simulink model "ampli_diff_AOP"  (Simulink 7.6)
settings: Solver=ode45  StartTime=0.0  StopTime=10.0  RelTol=1e-3
undefined symbols (not defined in the file or in its folder): Rb
libraries: fl_lib x16, nesl_utility x3

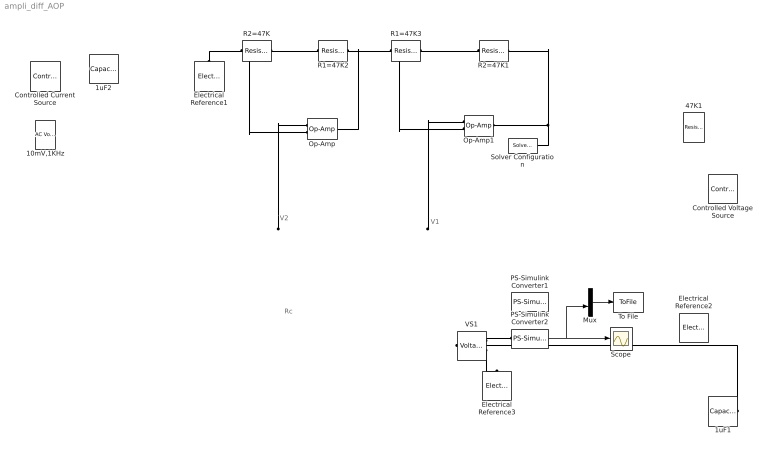
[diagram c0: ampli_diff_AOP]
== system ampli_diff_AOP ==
  note: Rc
  note: V2
  note: V1
  10mV,1KHz : fl_lib/Electrical/Electrical Sources/AC Voltage Source  DialogController=NetworkEngine.DynNeDlgSource  SystemSampleTime=-1  amp=0.01 V  shift=0 rad  omega=1000 Hz  i_Log=off  v_Log=off  LocalVarNames=|current|voltage|power  LocalVarDescs=|Current (A)|Voltage (V)|Power (W)  LocalVarLogging=[0 0 0]
  1uF1 : fl_lib/Electrical/Electrical Elements/Capacitor  DialogController=NetworkEngine.DynNeDlgSource  SystemSampleTime=-1  c=1e-06 F  v0=0 V  r=1e-06 Ohm  g=0 1/Ohm  i_Log=off  v_Log=off  vc_Log=off  LocalVarNames=|current|voltage|power  LocalVarDescs=|Capacitor current (A)|Voltage across capacitor (V)|Power (W)  LocalVarLogging=[0 0 0]
  1uF2 : fl_lib/Electrical/Electrical Elements/Capacitor  DialogController=NetworkEngine.DynNeDlgSource  SystemSampleTime=-1  c=1e-06 F  v0=0 V  r=1e-06 Ohm  g=0 1/Ohm  i_Log=off  v_Log=off  vc_Log=off  LocalVarNames=|current|voltage|power  LocalVarDescs=|Capacitor current (A)|Voltage across capacitor (V)|Power (W)  LocalVarLogging=[0 0 0]
  47K1 : fl_lib/Electrical/Electrical Elements/Resistor  DialogController=NetworkEngine.DynNeDlgSource  SystemSampleTime=-1  R=Rb Ohm  i_Log=off  v_Log=off  LocalVarNames=|current|voltage|power  LocalVarDescs=|Resistor current (A)|Voltage across resistor (V)|Power (W)  LocalVarLogging=[0 0 0]
  Controlled Current Source : fl_lib/Electrical/Electrical Sources/Controlled Current Source  DialogController=NetworkEngine.DynNeDlgSource  SystemSampleTime=-1  i_Log=off  v_Log=off  LocalVarNames=|i|v  LocalVarDescs=|i|v  LocalVarLogging=[0 0]
  Controlled Voltage Source : fl_lib/Electrical/Electrical Sources/Controlled Voltage Source  DialogController=NetworkEngine.DynNeDlgSource  SystemSampleTime=-1  i_Log=off  v_Log=off  LocalVarNames=|i|v  LocalVarDescs=|i|v  LocalVarLogging=[0 0]
  Electrical Reference1 : fl_lib/Electrical/Electrical Elements/Electrical Reference  DialogController=NetworkEngine.DynNeDlgSource  SystemSampleTime=-1  i_Log=off  LocalVarNames=|i  LocalVarDescs=|i  LocalVarLogging=[]
  Electrical Reference2 : fl_lib/Electrical/Electrical Elements/Electrical Reference  DialogController=NetworkEngine.DynNeDlgSource  SystemSampleTime=-1  i_Log=off  LocalVarNames=|i  LocalVarDescs=|i  LocalVarLogging=[]
  Electrical Reference3 : fl_lib/Electrical/Electrical Elements/Electrical Reference  DialogController=NetworkEngine.DynNeDlgSource  SystemSampleTime=-1  i_Log=off  LocalVarNames=|i  LocalVarDescs=|i  LocalVarLogging=[]
  Mux : Mux  Inputs=2
  Op-Amp : fl_lib/Electrical/Electrical Elements/Op-Amp  DialogController=NetworkEngine.DynNeDlgSource  SystemSampleTime=-1  i1_Log=off  v1_Log=off  outI_Log=off  LocalVarNames=|i1|v1|outI  LocalVarDescs=|i1|v1|outI  LocalVarLogging=[0 0 0]
  Op-Amp1 : fl_lib/Electrical/Electrical Elements/Op-Amp  DialogController=NetworkEngine.DynNeDlgSource  SystemSampleTime=-1  i1_Log=off  v1_Log=off  outI_Log=off  LocalVarNames=|i1|v1|outI  LocalVarDescs=|i1|v1|outI  LocalVarLogging=[0 0 0]
  PS-Simulink Converter1 : nesl_utility/PS-Simulink Converter  DialogController=NetworkEngine.DynNeUtilDlgSource  SystemSampleTime=-1  PhysicalDomain=network_engine_domain  LeftPortType=input  RightPortType=output  SubClassName=ps_output  Unit=1  AffineConversion=off
  PS-Simulink Converter2 : nesl_utility/PS-Simulink Converter  DialogController=NetworkEngine.DynNeUtilDlgSource  SystemSampleTime=-1  PhysicalDomain=network_engine_domain  LeftPortType=input  RightPortType=output  SubClassName=ps_output  Unit=1  AffineConversion=off
  R1=47K2 : fl_lib/Electrical/Electrical Elements/Resistor  DialogController=NetworkEngine.DynNeDlgSource  SystemSampleTime=-1  R=Rb Ohm  i_Log=off  v_Log=off  LocalVarNames=|current|voltage|power  LocalVarDescs=|Resistor current (A)|Voltage across resistor (V)|Power (W)  LocalVarLogging=[0 0 0]
  R1=47K3 : fl_lib/Electrical/Electrical Elements/Resistor  DialogController=NetworkEngine.DynNeDlgSource  SystemSampleTime=-1  R=Rb Ohm  i_Log=off  v_Log=off  LocalVarNames=|current|voltage|power  LocalVarDescs=|Resistor current (A)|Voltage across resistor (V)|Power (W)  LocalVarLogging=[0 0 0]
  R2=47K : fl_lib/Electrical/Electrical Elements/Resistor  DialogController=NetworkEngine.DynNeDlgSource  SystemSampleTime=-1  R=Rb Ohm  i_Log=off  v_Log=off  LocalVarNames=|current|voltage|power  LocalVarDescs=|Resistor current (A)|Voltage across resistor (V)|Power (W)  LocalVarLogging=[0 0 0]
  R2=47K1 : fl_lib/Electrical/Electrical Elements/Resistor  DialogController=NetworkEngine.DynNeDlgSource  SystemSampleTime=-1  R=Rb Ohm  i_Log=off  v_Log=off  LocalVarNames=|current|voltage|power  LocalVarDescs=|Resistor current (A)|Voltage across resistor (V)|Power (W)  LocalVarLogging=[0 0 0]
  Scope : Scope
  Solver Configuration : nesl_utility/Solver Configuration  DialogController=NetworkEngine.DynNeUtilDlgSource  SystemSampleTime=-1  PhysicalDomain=network_engine_domain  LeftPortType=input  RightPortType=generic  SubClassName=solver  Accelerate=off  Profile=off  ResidualTolerance=1e-9  MaxNonlinIter=12  MaxModeIter=2  DoFixedCost=off  UseLocalSampling=off  DoDC=off  LinearAlgebra=Sparse  LocalSolverSampleTime=.001  LocalSolverChoice=NE_BACKWARD_EULER_ADVANCER  UseLocalSolver=off
  To File : ToFile  Filename=es  MatrixName=x
  VS1 : fl_lib/Electrical/Electrical Sensors/Voltage Sensor  DialogController=NetworkEngine.DynNeDlgSource  SystemSampleTime=-1  i1_Log=off  v1_Log=off  LocalVarNames=|i1|v1  LocalVarDescs=|i1|v1  LocalVarLogging=[]
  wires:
  PS-Simulink Converter2/1 -> Mux/2, Scope/1
  Mux/1 -> To File/1
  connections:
  1uF1/RConn1 -- VS1/LConn1
  VS1/RConn2 -- Electrical Reference3/LConn1
  VS1/RConn1 -- PS-Simulink Converter2/LConn1
  Op-Amp/LConn1 -- ?
  Electrical Reference1/LConn1 -- R2=47K/LConn1
  R2=47K/RConn1 -- R1=47K2/LConn1 -- Op-Amp/LConn2
  R1=47K2/RConn1 -- R1=47K3/LConn1 -- Op-Amp/RConn1
  R1=47K3/RConn1 -- R2=47K1/LConn1 -- Op-Amp1/LConn2
  Op-Amp1/RConn1 -- R2=47K1/RConn1 -- Solver Configuration/RConn1
  Op-Amp1/LConn1 -- ?
